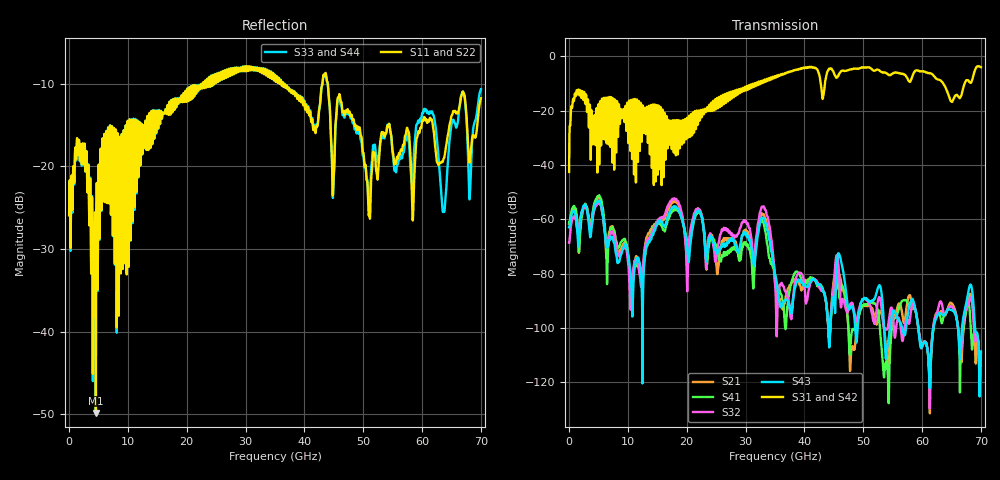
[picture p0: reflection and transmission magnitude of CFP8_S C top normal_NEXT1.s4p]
! AWR Design Environment (8415) Tue Jan 08 13:51:01 2019
! Document = 'CFP8 Channel_S_2'
! nPorts: 4, nXvals: 7001
# HZ S DB R 50
!Freq DBS11 AngS11 DBS12 AngS12 DBS13 AngS13 DBS14 AngS14
!	DBS21 AngS21 DBS22 AngS22 DBS23 AngS23 DBS24 AngS24
!	DBS31 AngS31 DBS32 AngS32 DBS33 AngS33 DBS34 AngS34
!	DBS41 AngS41 DBS42 AngS42 DBS43 AngS43 DBS44 AngS44
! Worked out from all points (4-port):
!   7000 points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, 10 MHz to 70 GHz, reference 50 ohm
!   strongest paths, dB at 10 MHz, 17.51 GHz, 35.01 GHz, 52.51 GHz, 70 GHz:
!     S31: -42.6, -29.7, -7.5, -4.9, -4.0
!     S42: -43.1, -29.6, -7.5, -4.9, -4.0
!     S43: -63.0, -55.5, -80.3, -85.2, -108.7
!     S32: -68.7, -52.5, -82.9, -89.9, -109.7
!     S41: -61.4, -56.9, -80.7, -94.0, -108.8
!     S21: -61.8, -53.8, -83.5, -96.7, -109.3
!   lowest |S11| = -49.9 dB at 4.56 GHz (marker M1), VSWR 1.01, Z = 50.3 + j0.11 ohm
!   |S11| at or under -10 dB: start of sweep to 22.77 GHz; 36.38 GHz to 43.06 GHz (6.686 GHz wide, 16.8 % of centre); 43.97 GHz to end of sweep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
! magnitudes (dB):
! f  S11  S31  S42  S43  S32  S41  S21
! 10 MHz  -25.9  -42.6  -43.1  -63.0  -68.7  -61.4  -61.8
! 4.56 GHz  -49.9  -23.7  -23.9  -54.0  -55.1  -52.6  -53.1
! 10.63 GHz  -14.4  -18.9  -18.9  -86.4  -85.5  -88.3  -90.5
! 17.86 GHz  -13.1  -29.4  -29.4  -55.2  -52.3  -56.4  -53.3
! 20.08 GHz  -10.8  -22.8  -23.0  -70.7  -86.6  -68.5  -79.9
! 32.97 GHz  -8.2  -9.1  -9.1  -59.6  -55.5  -61.2  -58.2
! 70 GHz  -11.8  -4.0  -4.0  -108.7  -109.7  -108.8  -109.3
